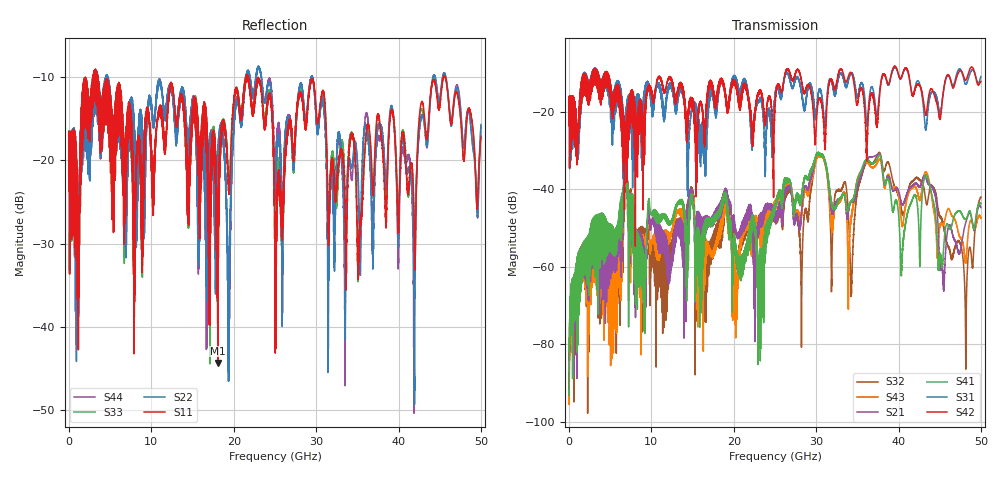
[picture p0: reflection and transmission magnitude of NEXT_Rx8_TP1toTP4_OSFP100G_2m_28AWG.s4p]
! Touchstone data
! Created: 27-Feb-2019 by IdEM 12 (12.1.0)
! COMMENTS
!  Created Wed Feb 27 12:03:36 2019
!  64 Port Network Data from SP1.SP block
!  freq  magS1_1  angS1_1  magS1_2  angS1_2  magS1_3  angS1_3  magS1_4  angS1_4
!  magS1_5  angS1_5  magS1_6  angS1_6  magS1_7  angS1_7  magS1_8  angS1_8
!  magS1_9  angS1_9  magS1_10  angS1_10  magS1_11  angS1_11  magS1_12  angS1_12
!  magS1_13  angS1_13  magS1_14  angS1_14  magS1_15  angS1_15  magS1_16  angS1_16
!  magS1_17  angS1_17  magS1_18  angS1_18  magS1_19  angS1_19  magS1_20  angS1_20
!  magS1_21  angS1_21  magS1_22  angS1_22  magS1_23  angS1_23  magS1_24  angS1_24
!  magS1_25  angS1_25  magS1_26  angS1_26  magS1_27  angS1_27  magS1_28  angS1_28
!  magS1_29  angS1_29  magS1_30  angS1_30  magS1_31  angS1_31  magS1_32  angS1_32
!  magS1_33  angS1_33  magS1_34  angS1_34  magS1_35  angS1_35  magS1_36  angS1_36
!  magS1_37  angS1_37  magS1_38  angS1_38  magS1_39  angS1_39  magS1_40  angS1_40
!  magS1_41  angS1_41  magS1_42  angS1_42  magS1_43  angS1_43  magS1_44  angS1_44
!  magS1_45  angS1_45  magS1_46  angS1_46  magS1_47  angS1_47  magS1_48  angS1_48
!  magS1_49  angS1_49  magS1_50  angS1_50  magS1_51  angS1_51  magS1_52  angS1_52
!  magS1_53  angS1_53  magS1_54  angS1_54  magS1_55  angS1_55  magS1_56  angS1_56
!  magS1_57  angS1_57  magS1_58  angS1_58  magS1_59  angS1_59  magS1_60  angS1_60
!  magS1_61  angS1_61  magS1_62  angS1_62  magS1_63  angS1_63  magS1_64  angS1_64
!  magS2_1  angS2_1  magS2_2  angS2_2  magS2_3  angS2_3  magS2_4  angS2_4
!  magS2_5  angS2_5  magS2_6  angS2_6  magS2_7  angS2_7  magS2_8  angS2_8
!  magS2_9  angS2_9  magS2_10  angS2_10  magS2_11  angS2_11  magS2_12  angS2_12
!  magS2_13  angS2_13  magS2_14  angS2_14  magS2_15  angS2_15  magS2_16  angS2_16
!  magS2_17  angS2_17  magS2_18  angS2_18  magS2_19  angS2_19  magS2_20  angS2_20
!  magS2_21  angS2_21  magS2_22  angS2_22  magS2_23  angS2_23  magS2_24  angS2_24
!  magS2_25  angS2_25  magS2_26  angS2_26  magS2_27  angS2_27  magS2_28  angS2_28
!  magS2_29  angS2_29  magS2_30  angS2_30  magS2_31  angS2_31  magS2_32  angS2_32
!  magS2_33  angS2_33  magS2_34  angS2_34  magS2_35  angS2_35  magS2_36  angS2_36
!  magS2_37  angS2_37  magS2_38  angS2_38  magS2_39  angS2_39  magS2_40  angS2_40
!  magS2_41  angS2_41  magS2_42  angS2_42  magS2_43  angS2_43  magS2_44  angS2_44
!  magS2_45  angS2_45  magS2_46  angS2_46  magS2_47  angS2_47  magS2_48  angS2_48
!  magS2_49  angS2_49  magS2_50  angS2_50  magS2_51  angS2_51  magS2_52  angS2_52
!  magS2_53  angS2_53  magS2_54  angS2_54  magS2_55  angS2_55  magS2_56  angS2_56
!  magS2_57  angS2_57  magS2_58  angS2_58  magS2_59  angS2_59  magS2_60  angS2_60
!  magS2_61  angS2_61  magS2_62  angS2_62  magS2_63  angS2_63  magS2_64  angS2_64
!  magS3_1  angS3_1  magS3_2  angS3_2  magS3_3  angS3_3  magS3_4  angS3_4
!  magS3_5  angS3_5  magS3_6  angS3_6  magS3_7  angS3_7  magS3_8  angS3_8
!  magS3_9  angS3_9  magS3_10  angS3_10  magS3_11  angS3_11  magS3_12  angS3_12
!  magS3_13  angS3_13  magS3_14  angS3_14  magS3_15  angS3_15  magS3_16  angS3_16
!  magS3_17  angS3_17  magS3_18  angS3_18  magS3_19  angS3_19  magS3_20  angS3_20
!  magS3_21  angS3_21  magS3_22  angS3_22  magS3_23  angS3_23  magS3_24  angS3_24
!  magS3_25  angS3_25  magS3_26  angS3_26  magS3_27  angS3_27  magS3_28  angS3_28
!  magS3_29  angS3_29  magS3_30  angS3_30  magS3_31  angS3_31  magS3_32  angS3_32
!  magS3_33  angS3_33  magS3_34  angS3_34  magS3_35  angS3_35  magS3_36  angS3_36
!  magS3_37  angS3_37  magS3_38  angS3_38  magS3_39  angS3_39  magS3_40  angS3_40
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# Hz S MA R 50
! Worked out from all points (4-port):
!   5000 points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, 10 MHz to 50 GHz, reference 50 ohm
!   strongest paths, dB at 10 MHz, 12.51 GHz, 25.01 GHz, 37.51 GHz, 50 GHz:
!     S42: -18.0, -12.2, -18.3, -20.7, -12.2
!     S31: -18.0, -14.0, -15.8, -18.9, -11.0
!     S41: -92.0, -47.8, -44.8, -31.8, -43.7
!     S21: -93.1, -56.7, -47.8, -31.1, -44.8
!     S43: -94.2, -50.5, -45.0, -32.8, -47.5
!     S32: -93.9, -54.2, -48.1, -30.8, -42.1
!   lowest |S11| = -44.3 dB at 18.09 GHz (marker M1), VSWR 1.01, Z = 49.5 + j0.362 ohm
!   |S11| at or under -10 dB: 3.49 GHz to 21.47 GHz (17.98 GHz wide, 144 % of centre); 21.77 GHz to 45.47 GHz (23.7 GHz wide, 70.5 % of centre); 45.66 GHz to end of sweep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
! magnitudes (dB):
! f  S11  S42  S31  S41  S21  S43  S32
! 10 MHz  -17.7  -18.0  -18.0  -92.0  -93.1  -94.2  -93.9
! 6.9 GHz  -25.7  -28.0  -29.4  -33.1  -34.7  -35.3  -37.1
! 18.09 GHz  -44.3  -15.3  -16.7  -47.4  -46.7  -53.9  -50.7
! 34.3 GHz  -16.8  -10.1  -10.2  -43.3  -43.3  -47.0  -64.7
! 37.63 GHz  -15.0  -17.5  -16.3  -31.3  -31.1  -32.4  -30.5
! 48.14 GHz  -17.5  -11.9  -12.9  -47.8  -48.8  -58.7  -77.1
! 50 GHz  -17.2  -12.2  -11.0  -43.7  -44.8  -47.5  -42.1
